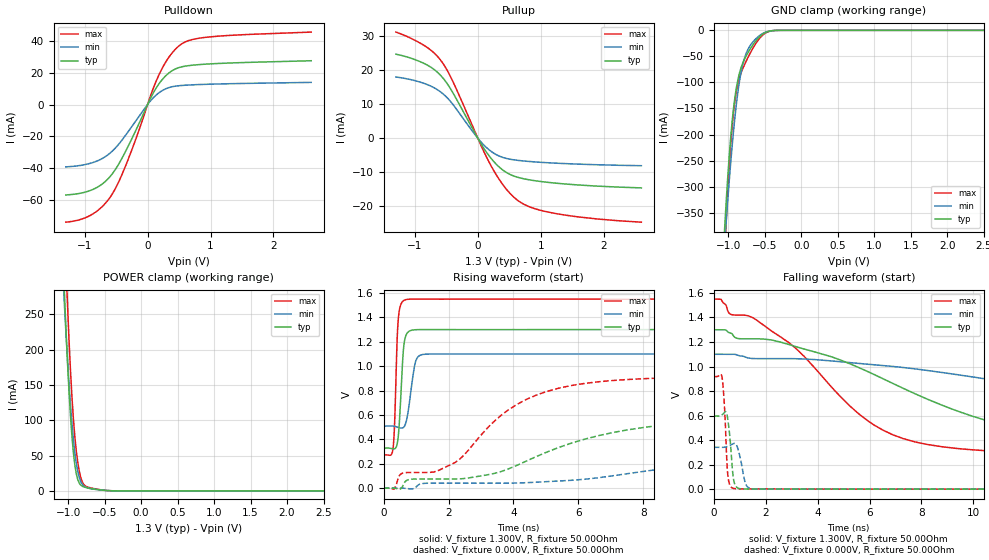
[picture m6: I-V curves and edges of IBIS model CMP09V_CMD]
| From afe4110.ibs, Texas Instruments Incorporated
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|   CMP09V_CMD  model
[Model]   CMP09V_CMD
Model_type   I/O
Vinl =  0.39V |0.275V for 1.1V
Vinh =  0.91V |0.825V for 1.1V
Vmeas = 1.500V
Cref = 25pF |25pF for VDD=1.55V; 15pF for VDD=1.1V
|   typ   min   max
|   (nom)   (fast)   (weak)
C_comp   0.8824pF   0.8662pF   0.9071pF
[Model Spec]
Vinl   0.39V   0.275V   0.465V
Vinh   0.91V   0.825V   1.085V
[Voltage Range]   1.300V   1.100V   1.550V
[Temperature Range]   27.0   85.0   0.0
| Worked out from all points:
|   slope of the pulldown table from 0 to 0.195 V, typ, clamps not added: 14.2 ohm
|   slope of the pullup table from 0 to 0.195 V, typ, clamps not added: 34.9 ohm
|   GND clamp passes 1 mA (typ) near -0.42 V on its own axis
|   POWER clamp passes 1 mA (typ) near -0.52 V on its own axis
|   falling waveform, V_fixture 1.300V, R_fixture 50.00Ohm: 20-80 % time 7.04ns typ, 13.5ns min, 3.95ns max; typ from 1.3 V to 0.329 V
|   rising waveform, V_fixture 1.300V, R_fixture 50.00Ohm: 20-80 % time 121ps typ, 185ps min, 91.9ps max; typ from 0.329 V to 1.3 V
|   rising waveform, V_fixture 0.000V, R_fixture 50.00Ohm: 20-80 % time 4.12ns typ, 7.41ns min, 2.47ns max; typ from 0 V to 0.596 V
|   falling waveform, V_fixture 0.000V, R_fixture 50.00Ohm: 20-80 % time 143ps typ, 193ps min, 121ps max; typ from 0.596 V to 0 V
[Pulldown]
|   Voltage   I(typ)   I(min)   I(max)
-1.3V     -56.75mA   -39.13mA   -73.85mA
-888.4mV  -53.62mA   -36.64mA   -69.09mA
-712.1mV  -49.6mA    -33.68mA   -63.7mA
-574.9mV  -44.18mA   -29.74mA   -56.96mA
-457.3mV  -37.25mA   -24.83mA   -48.37mA
-320.1mV  -27.06mA   -17.66mA   -35.55mA
150.3mV   11.21mA    6.413mA    15.97mA
326.6mV   19.39mA    10.45mA    29mA
522.6mV   23.44mA    11.87mA    37.5mA
718.6mV   24.69mA    12.35mA    40.85mA
1.032V    25.56mA    12.78mA    42.57mA
2.6V      27.46mA    13.88mA    45.44mA
[GND Clamp]
|   Voltage   I(typ)   I(min)   I(max)
-1.3V     -1.155A    -1.095A    -1.249A
-1.065V   -415.4mA   -439.7mA   -467.4mA
-1.045V   -365.6mA   -398.1mA   -410.2mA
-1.026V   -319.2mA   -358.7mA   -355.9mA
-966.8mV  -203.4mA   -252.2mA   -218mA
-927.6mV  -147.8mA   -191mA     -154.9mA
-868.8mV  -94.41mA   -117.6mA   -102mA
-810.1mV  -65.43mA   -69.87mA   -76.07mA
-751.3mV  -47.8mA    -42.62mA   -57.78mA
-555.3mV  -10.16mA   -8.413mA   -12.64mA
-320.1mV  -77.94uA   -90.57uA   -96.79uA
2.6V      0A         0A         0A
[Pullup]
|   Voltage   I(typ)   I(min)   I(max)
-1.3V     24.77mA    18.03mA    31.28mA
-829.6mV  21.82mA    15.98mA    27.07mA
-672.9mV  19.94mA    14.63mA    24.76mA
-555.3mV  17.78mA    13.11mA    22.12mA
-378.9mV  12.86mA    9.547mA    16.05mA
0V        193.7nA    138.7nA    226.6nA
169.8mV   -4.968mA   -3.301mA   -6.724mA
405mV     -9.522mA   -5.753mA   -13.91mA
620.6mV   -11.49mA   -6.541mA   -18.18mA
855.8mV   -12.44mA   -6.966mA   -20.53mA
1.209V    -13.25mA   -7.378mA   -22.18mA
2.6V      -14.71mA   -8.161mA   -24.83mA
[POWER Clamp]
|   Voltage   I(typ)   I(min)   I(max)
-1.3V     1.028A     926mA      1.167A
-1.065V   317.2mA    292.9mA    417.5mA
-1.045V   267.1mA    253mA      361.7mA
-1.026V   220.1mA    215.8mA    308.1mA
-1.006V   177mA      181.2mA    257.6mA
-966.8mV  105mA      120.5mA    168.9mA
-927.6mV  54.19mA    72.67mA    101.7mA
-868.8mV  16.35mA    28.04mA    41.23mA
-810.1mV  6.868mA    9.986mA    13.71mA
-731.7mV  4.215mA    4.108mA    5.448mA
-398.5mV  154.7uA    187.5uA    190.9uA
2.6V      -36.78uA   -23.84uA   -58.74uA
[Ramp]
R_load = 50.00Ohm
|   typ   min   max
dV/dt_r   357.465mV/4.118ns   204.669mV/7.411ns   550.571mV/2.451ns
dV/dt_f   582.793mV/7.031ns   354.279mV/13.446ns  766.389mV/3.946ns
[Falling Waveform]
V_fixture = 1.300V
V_fixture_min = 1.100V
V_fixture_max = 1.550V
R_fixture = 50.00Ohm
|   Time   V(typ)   V(min)   V(max)
0s        1.3V       1.1V       1.55V
640ps     1.273V     1.1V       1.427V
2.91ns    1.178V     1.064V     1.192V
5.25ns    1.022V     1.032V     677.1mV
6.5ns     902.4mV    1.008V     483.5mV
8.27ns    730.4mV    966.6mV    363.2mV
11.13ns   524.1mV    877.9mV    305.8mV
17.32ns   370.3mV    699.9mV    277.7mV
32.9ns    329.3mV    533.2mV    272.5mV
125ns     328.7mV    509.5mV    272.7mV
[Rising Waveform]
V_fixture = 1.300V
V_fixture_min = 1.100V
V_fixture_max = 1.550V
R_fixture = 50.00Ohm
|   Time   V(typ)   V(min)   V(max)
0s        328.7mV    509.5mV    272.7mV
290ps     323mV      509mV      327mV
340ps     323.7mV    506.3mV    550.5mV
420ps     366.5mV    500.3mV    1.246V
490ps     565.6mV    495.4mV    1.466V
620ps     1.163V     500.3mV    1.538V
810ps     1.29V      734.1mV    1.549V
1.01ns    1.299V     1.056V     1.55V
1.43ns    1.3V       1.099V     1.549V
125ns     1.3V       1.1V       1.55V
[Rising Waveform]
V_fixture = 0.000V
V_fixture_min = 0.000V
V_fixture_max = 0.000V
R_fixture = 50.00Ohm
|   Time   V(typ)   V(min)   V(max)
0s        388.9uV    395.4uV    454.7uV
320ps     217.8uV    545.3uV    -7.874mV
580ps     13.86mV    191.2uV    122.6mV
2.19ns    75.24mV    41.28mV    209mV
3.58ns    133.2mV    41.15mV    588mV
4.69ns    257.6mV    48.98mV    761.3mV
8.78ns    522.5mV    164.9mV    904.8mV
14.86ns   588.7mV    292.4mV    918.3mV
23.33ns   596.4mV    334.6mV    918.2mV
125ns     596.2mV    341.5mV    918.1mV
[Falling Waveform]
V_fixture = 0.000V
V_fixture_min = 0.000V
V_fixture_max = 0.000V
R_fixture = 50.00Ohm
|   Time   V(typ)   V(min)   V(max)
0s        596.2mV    341.5mV    918.1mV
320ps     607.1mV    341.3mV    909.8mV
410ps     624.9mV    342.2mV    680.3mV
490ps     620.8mV    345.9mV    291.6mV
600ps     466.9mV    354.9mV    44.82mV
750ps     97.62mV    370.7mV    7.093mV
920ps     10.84mV    335.1mV    3.41mV
1.25ns    1.681mV    33.21mV    2.702mV
1.68ns    1.781mV    1.419mV    2.591mV
125ns     388.9uV    395.4uV    454.7uV
